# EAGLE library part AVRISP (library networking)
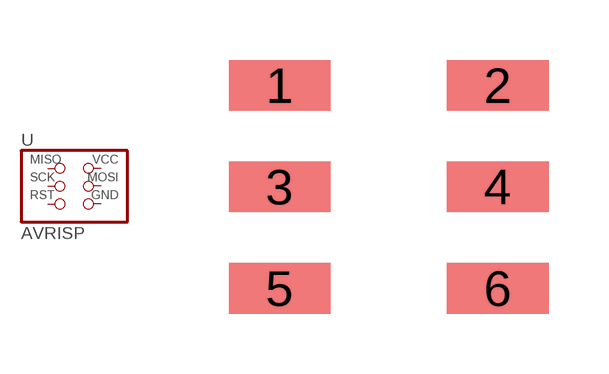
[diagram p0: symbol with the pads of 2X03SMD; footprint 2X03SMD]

Designator prefix -

## AVRISPSMD  [2X03SMD]
1  MISO  pas
2  VCC  pas
3  SCK  pas
4  MOSI  pas
5  RST  pas
6  GND  pas

## Footprint 2X03SMD (pad centres in mm)
smd 2.54 x 1.27: 1 -2.54,2.54; 2 2.92,2.54; 3 -2.54,0; 4 2.92,0; 5 -2.54,-2.54; 6 2.92,-2.54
